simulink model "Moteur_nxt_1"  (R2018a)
settings: Solver=FixedStepAuto  StartTime=0.0  StopTime=inf  RelTol=1e-3  EnableMultiTasking=on
libraries: arduinolib x3, simulink x1

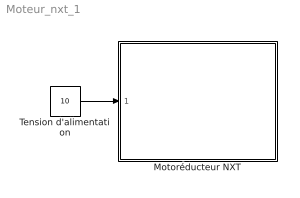
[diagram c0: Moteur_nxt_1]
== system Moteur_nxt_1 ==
  Motoréducteur NXT : Subsystem
  Tension d'alimentation : Constant  Value=10
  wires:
  Tension d'alimentation/1 -> Motoréducteur NXT/1(U)

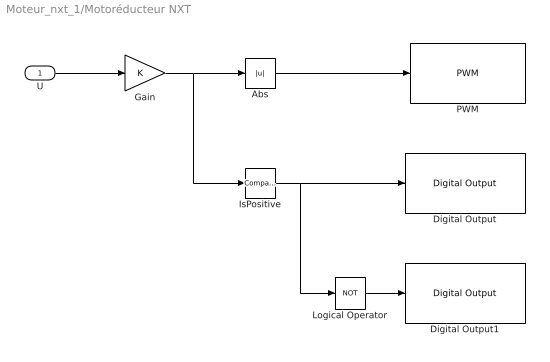
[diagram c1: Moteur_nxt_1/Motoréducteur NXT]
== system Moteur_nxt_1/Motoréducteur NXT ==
  U : Inport
  Abs : Abs
  Digital Output : arduinolib/Digital Output  pinNumber=3  blockPlatform=arduino
  Digital Output1 : arduinolib/Digital Output  pinNumber=3  blockPlatform=arduino
  Gain : Gain
  IsPositive : simulink/Logic and Bit Operations/Compare To Zero  relop=>  OutDataTypeStr=boolean
  Logical Operator : Logic  Operator=NOT  AllPortsSameDT=off  OutDataTypeStr=boolean
  PWM : arduinolib/PWM  pinNumber=3  EnableInputFrequency=off  InitialFrequency=2000  InitialDutyCycle=0  NotificationType=None  blockPlatform=arduino
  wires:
  IsPositive/1 -> Logical Operator/1, Digital Output/1
  U/1 -> Gain/1
  Gain/1 -> IsPositive/1, Abs/1
  Abs/1 -> PWM/1
  Logical Operator/1 -> Digital Output1/1
